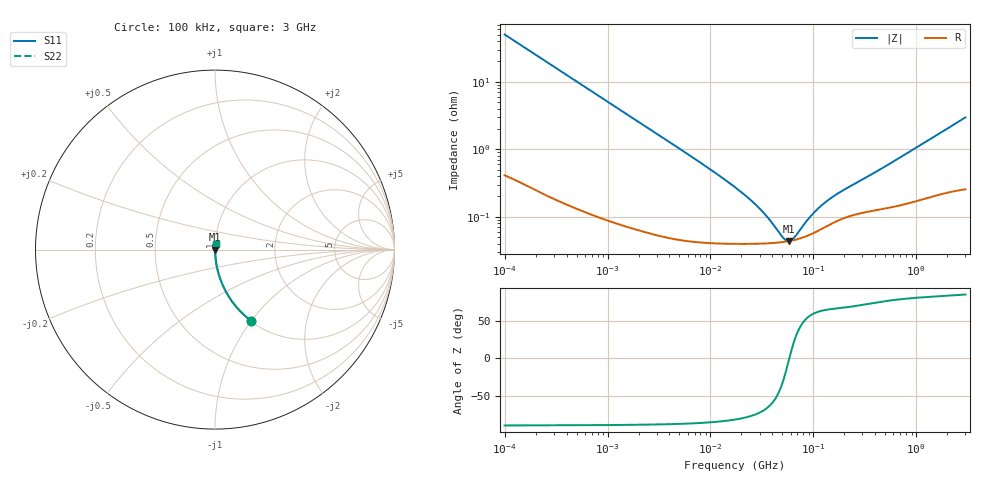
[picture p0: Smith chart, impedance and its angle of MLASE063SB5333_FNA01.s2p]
! MLASE063SB5333_FNA01  S-PARAMETER MODEL  ( Standard Model )
! Model Generated by TAIYO YUDEN Corporation (http://www.ty-top.com)
! Version 1.0
! TAIYO YUDEN Control No. 220601
! Copyright(c) 2013 TAIYO YUDEN CO.,LTD. All Rights Reserved.
! Product Description (link to TY-COMPAS)
! https://ds.yuden.co.jp/TYCOMPAS/or/detail?pn=MLASE063SB5333KFNA01&u=M
! Products Name : Multilayer Ceramic Capacitors
! Characteristics :
!  Capacitance : 0.033 [uF] , Rated Voltage : 16 [V] , TCC : X5R
!  Case Size : 0.6 x 0.3 / 0.024 x 0.012 [mm/inch] , Thickness : 0.3 / 0.012 [mm/inch]
!  (Conditions: Temperature = 25 [degC] , DC Bias Voltage = 0 [V])
! External Node Assignments :
!  1  o---| |---o  2
! GND o---------o GND
! Frequency Range : 100kHz  -  3GHz  [ 401 STEP ]
# MHZ S RI R 50
! Freq[MHz].  S11 Real  S11 Imag  S21 Real  S21 Imag  S12 Real  S12 Imag  S22 Real  S22 Imag
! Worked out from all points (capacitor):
!   401 points, 100 kHz to 3 GHz, reference 50 ohm
!   read as one part in series: C = 31.7 nF near 105.3 kHz
!   lowest |Z| = 43.7 mohm at 58.16 MHz (marker M1)
!   series resonance near 58.4 MHz, so ESL is about 230 pH
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0.1  0.2027 -0.3979  0.7973 0.3979  0.7973 0.3979  0.2027 -0.3979
0.14345  0.1114 -0.3101  0.8886 0.3101  0.8886 0.3101  0.1114 -0.3101
0.205778  0.0585 -0.2297  0.9415 0.2297  0.9415 0.2297  0.0585 -0.2297
0.335785  0.0237 -0.1465  0.9763 0.1465  0.9763 0.1465  0.0237 -0.1465
0.562235  0.00923 -0.0891  0.9908 0.0891  0.9908 0.0891  0.00923 -0.0891
1.18716  0.00263 -0.0427  0.9974 0.0427  0.9974 0.0427  0.00263 -0.0427
3.161081  0.000784 -0.0161  0.9992 0.0161  0.9992 0.0161  0.000784 -0.0161
9.331111  0.000438 -0.00537  0.9996 0.00537  0.9996 0.00537  0.000438 -0.00537
17.7727  0.000404 -0.00263  0.9996 0.00263  0.9996 0.00263  0.000404 -0.00263
22.99754  0.0004 -0.00189  0.9996 0.00189  0.9996 0.00189  0.0004 -0.00189
29.00125  0.000401 -0.00134  0.9996 0.00134  0.9996 0.00134  0.000401 -0.00134
36.57227  0.000406 -0.000858  0.9996 0.000858  0.9996 0.000858  0.000406 -0.000858
51.12795  0.000424 -0.000236  0.9996 0.000236  0.9996 0.000236  0.000424 -0.000236
55.23785  0.000431 -9.84e-05  0.9996 9.84e-05  0.9996 9.84e-05  0.000431 -9.84e-05
58.15973  0.000437 -7.15e-06  0.9996 7.15e-06  0.9996 7.15e-06  0.000437 -7.15e-06
61.23616  0.000444 8.4e-05  0.9996 -8.4e-05  0.9996 -8.4e-05  0.000444 8.4e-05
66.15861  0.000456 0.000221  0.9995 -0.000221  0.9995 -0.000221  0.000456 0.000221
97.38194  0.000562 0.000922  0.9994 -0.000922  0.9994 -0.000922  0.000562 0.000922
122.8043  0.000673 0.00136  0.9993 -0.00136  0.9993 -0.00136  0.000673 0.00136
163.0551  0.000843 0.00191  0.9992 -0.00191  0.9992 -0.00191  0.000843 0.00191
547.5153  0.0014 0.00589  0.9986 -0.00589  0.9986 -0.00589  0.0014 0.00589
3000  0.00341 0.0294  0.9966 -0.0294  0.9966 -0.0294  0.00341 0.0294
